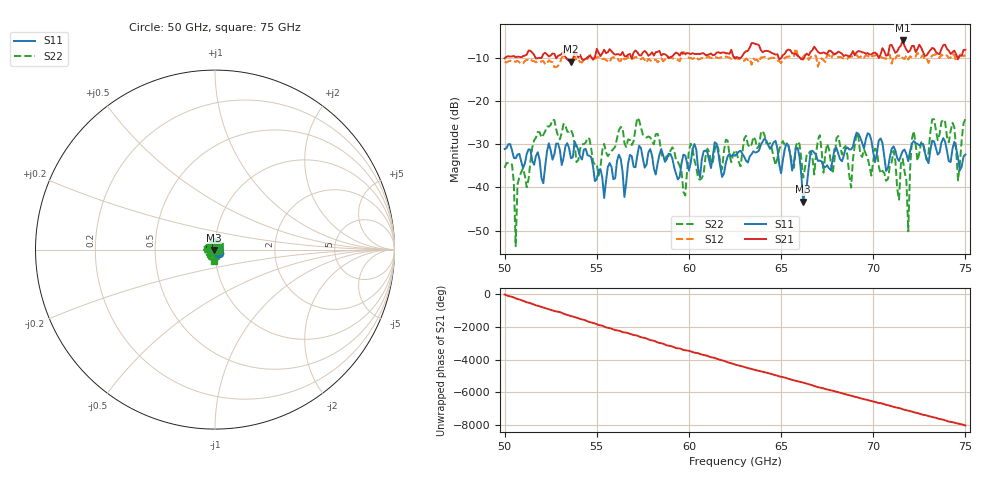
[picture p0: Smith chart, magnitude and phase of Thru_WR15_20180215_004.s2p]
# GHz S RI R 50
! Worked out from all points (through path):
!   251 points, 50 GHz to 75 GHz, reference 50 ohm
!   highest |S21| = -5.97 dB at 71.6 GHz (marker M1); lowest = -10.9 dB at 53.6 GHz (marker M2)
!   lowest |S11| = -43.3 dB at 66.2 GHz (marker M3), VSWR 1.01, Z = 49.3 - j0.138 ohm
!   |S11| at or under -10 dB: start of sweep to end of sweep
!   |S22| runs from -53.6 to -23.9 dB; largest |S21 - S12| = 0.78
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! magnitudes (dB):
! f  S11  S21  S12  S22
! 50 GHz  -31.1  -10.1  -11.0  -35.5
! 50.4 GHz  -31.4  -9.6  -10.8  -34.7
! 50.6 GHz  -33.3  -9.8  -10.9  -53.6
! 50.7 GHz  -32.4  -9.7  -10.7  -39.3
! 51.8 GHz  -31.8  -10.1  -10.8  -27.2
! 53.6 GHz  -33.3  -10.9  -10.6  -26.7
! 54.2 GHz  -33.5  -10.3  -11.1  -30.0
! 56.5 GHz  -42.2  -9.6  -10.3  -29.7
! 58.4 GHz  -32.4  -8.4  -10.7  -28.8
! 59.8 GHz  -32.6  -9.0  -8.9  -41.9
! 60.1 GHz  -34.2  -9.1  -10.0  -29.9
! 62.5 GHz  -32.7  -10.2  -9.8  -31.3
! 65.9 GHz  -30.8  -9.6  -9.3  -29.4
! 66.2 GHz  -43.3  -10.4  -9.8  -37.7
! 66.7 GHz  -31.5  -8.2  -9.5  -33.0
! 70.9 GHz  -33.1  -7.1  -9.3  -35.0
! 71.6 GHz  -31.6  -6.0  -10.1  -33.4
! 71.9 GHz  -33.9  -8.7  -10.4  -50.2
! 72.2 GHz  -29.2  -7.2  -9.7  -26.9
! 74.3 GHz  -31.0  -8.7  -9.1  -25.0
! 74.6 GHz  -33.1  -10.2  -10.3  -38.4
! 75 GHz  -32.4  -8.1  -9.4  -24.1
